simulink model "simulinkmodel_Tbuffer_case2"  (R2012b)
settings: Solver=ode3  StartTime=0.0  StopTime=3600*24  FixedStep=60  RelTol=1e-12
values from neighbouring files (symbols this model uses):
  Pthreshold = Pricethresholdvector(1)    [cost_general_case1.m]
  qinlb = qin_min    (= 0)    [objective_generall.m]
  qinub = qin_max    (= 10)    [objective_generall.m]
  Qlb = Qmin    (= 0)    [objective_generall.m]
  Qub = Qmax    (= 5.5)    [objective_generall.m]
libraries: simulink x2

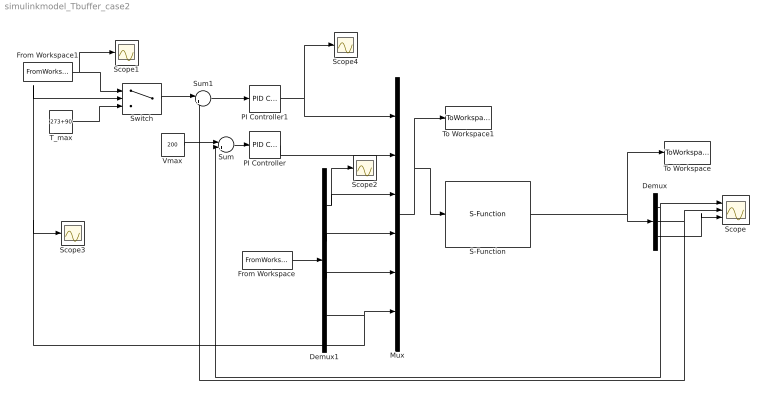
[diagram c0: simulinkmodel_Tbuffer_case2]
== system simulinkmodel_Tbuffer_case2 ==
  Demux : Demux  Outputs=3
  Demux1 : Demux
  From Workspace : FromWorkspace  VariableName=dsim  SampleTime=0  OutputAfterFinalValue=Setting to zero
  From Workspace1 : FromWorkspace  VariableName=Tbuffer  SampleTime=0  Interpolate=off  OutputAfterFinalValue=Holding final value
  Mux : Mux  Inputs=6
  PI Controller : simulink/Continuous/PID Controller  Controller=PI  TimeDomain=Continuous-time  SampleTime=1  IntegratorMethod=Forward Euler  FilterMethod=Forward Euler  Form=Ideal  P=3  I=1/80  D=0  N=100  InitialConditionSource=internal  InitialConditionForIntegrator=0  InitialConditionForFilter=0  ExternalReset=none  LimitOutput=on  UpperSaturationLimit=qinub  LowerSaturationLimit=qinlb  LinearizeAsGain=on  AntiWindupMode=clamping  Kb=1  TrackingMode=off  Kt=1  PParamMin=[]  PParamMax=[]  IParamMin=[]  IParamMax=[]  DParamMin=[]  DParamMax=[]  NParamMin=[]  NParamMax=[]  KbParamMin=[]  KbParamMax=[]  KtParamMin=[]  KtParamMax=[]  POutMin=[]  POutMax=[]  IOutMin=[]  IOutMax=[]  DOutMin=[]  DOutMax=[]  NOutMin=[]  NOutMax=[]  KbOutMin=[]  KbOutMax=[]  KtOutMin=[]  KtOutMax=[]  IntegratorOutMin=[]  IntegratorOutMax=[]  FilterOutMin=[]  FilterOutMax=[]  SumOutMin=[]  SumOutMax=[]  SumI1OutMin=[]  SumI1OutMax=[]  SumI2OutMin=[]  SumI2OutMax=[]  SumI3OutMin=[]  SumI3OutMax=[]  SumDOutMin=[]  SumDOutMax=[]  SaturationOutMin=[]  SaturationOutMax=[]  IntegratorContinuousStateAttributes=''  IntegratorStateMustResolveToSignalObject=off  IntegratorRTWStateStorageClass=Auto  FilterContinuousStateAttributes=''  FilterStateMustResolveToSignalObject=off  FilterRTWStateStorageClass=Auto
  PI Controller1 : simulink/Continuous/PID Controller  Controller=PI  TimeDomain=Continuous-time  SampleTime=1  IntegratorMethod=Forward Euler  FilterMethod=Forward Euler  Form=Ideal  P=50  I=1/80  D=0  N=100  InitialConditionSource=internal  InitialConditionForIntegrator=0  InitialConditionForFilter=0  ExternalReset=none  LimitOutput=on  UpperSaturationLimit=Qub  LowerSaturationLimit=Qlb  LinearizeAsGain=on  AntiWindupMode=clamping  Kb=1  TrackingMode=off  Kt=1  PParamMin=[]  PParamMax=[]  IParamMin=[]  IParamMax=[]  DParamMin=[]  DParamMax=[]  NParamMin=[]  NParamMax=[]  KbParamMin=[]  KbParamMax=[]  KtParamMin=[]  KtParamMax=[]  POutMin=[]  POutMax=[]  IOutMin=[]  IOutMax=[]  DOutMin=[]  DOutMax=[]  NOutMin=[]  NOutMax=[]  KbOutMin=[]  KbOutMax=[]  KtOutMin=[]  KtOutMax=[]  IntegratorOutMin=[]  IntegratorOutMax=[]  FilterOutMin=[]  FilterOutMax=[]  SumOutMin=[]  SumOutMax=[]  SumI1OutMin=[]  SumI1OutMax=[]  SumI2OutMin=[]  SumI2OutMax=[]  SumI3OutMin=[]  SumI3OutMax=[]  SumDOutMin=[]  SumDOutMax=[]  SaturationOutMin=[]  SaturationOutMax=[]  IntegratorContinuousStateAttributes=''  IntegratorStateMustResolveToSignalObject=off  IntegratorRTWStateStorageClass=Auto  FilterContinuousStateAttributes=''  FilterStateMustResolveToSignalObject=off  FilterRTWStateStorageClass=Auto
  S-Function : S-Function  FunctionName=sfunctionmodel  Parameters=par  EnableBusSupport=off
  Scope : Scope  NumInputPorts=3
  Scope{1..4} (4 alike) : Scope
  Sum : Sum  Inputs=|+-
  Sum1 : Sum  Inputs=|+-
  Switch : Switch  Threshold=Pthreshold
  T_max : Constant  Value=273+90
  To Workspace : ToWorkspace  VariableName=simout  SampleTime=-1
  To Workspace1 : ToWorkspace  VariableName=u  SampleTime=-1  SaveFormat=Structure With Time
  Vmax : Constant  Value=200
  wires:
  Mux/1 -> To Workspace1/1, S-Function/1
  Demux/1 -> Sum/2, Scope/1
  Demux/2 -> Scope/2, Sum1/2
  Vmax/1 -> Sum/1
  Sum/1 -> PI Controller/1
  PI Controller/1 -> Mux/2
  S-Function/1 -> To Workspace/1, Demux/1
  Sum1/1 -> PI Controller1/1
  PI Controller1/1 -> Scope4/1, Mux/1
  From Workspace/1 -> Demux1/1
  Demux1/1 -> Scope2/1, Mux/3
  Demux1/2 -> Mux/4
  Demux1/3 -> Mux/5
  Demux1/4 -> Scope3/1, Switch/2, Mux/6
  Demux/3 -> Scope/3
  Switch/1 -> Sum1/1
  T_max/1 -> Switch/3
  From Workspace1/1 -> Scope1/1, Switch/1
